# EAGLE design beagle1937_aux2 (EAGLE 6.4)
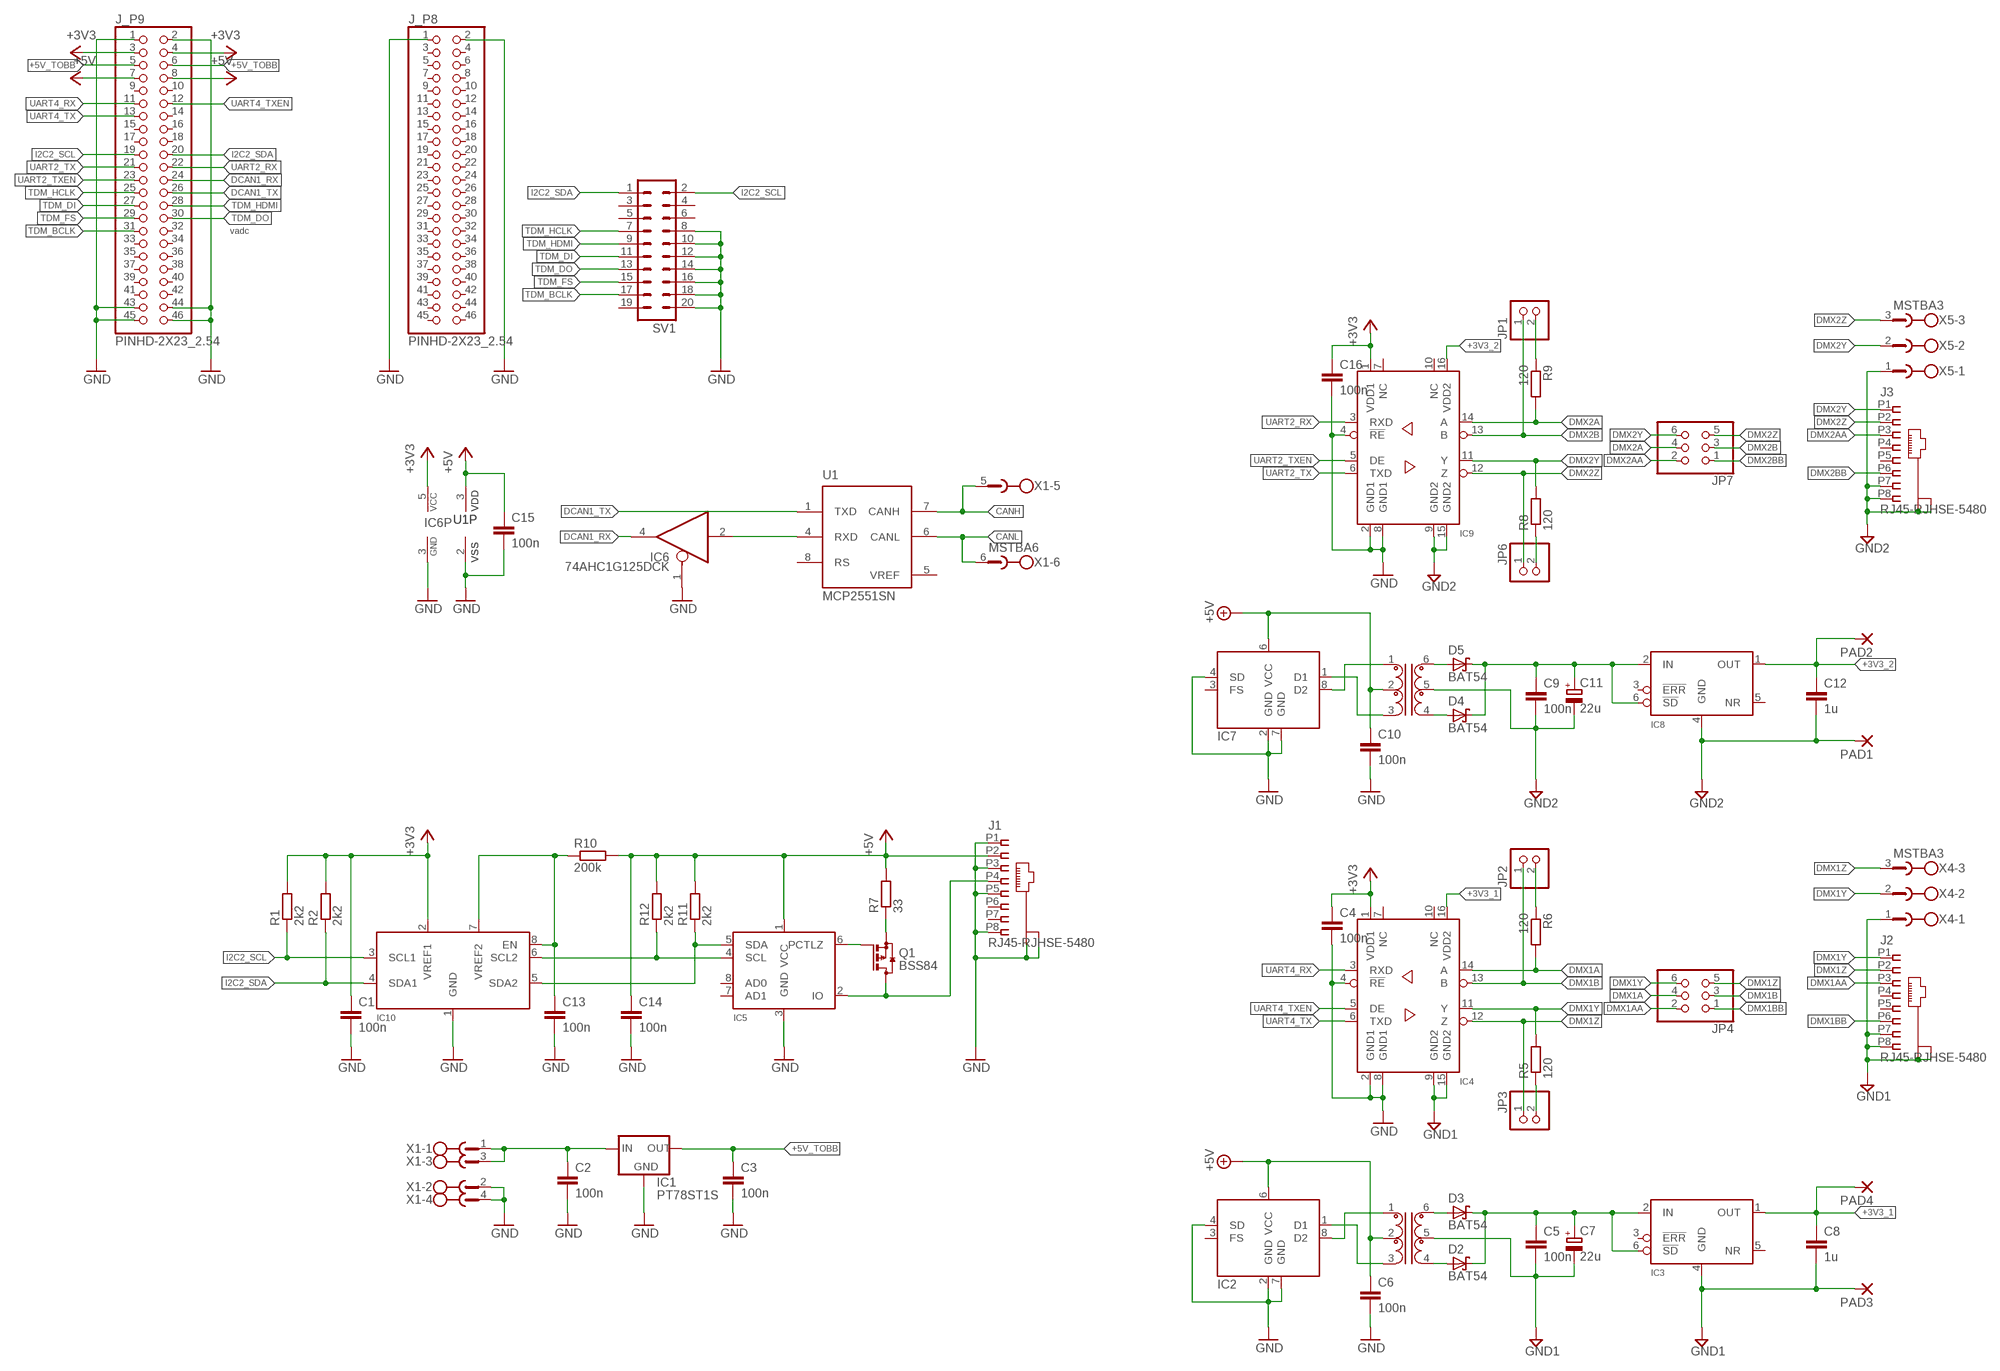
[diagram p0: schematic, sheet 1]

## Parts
C1  100n  C-EUC0603  [C0603]
C2  100n  C-EUC0603  [C0603]
C3  100n  C-EUC0603  [C0603]
C4  100n  C-EUC0603  [C0603]
C5  100n  C-EUC0603  [C0603]
C6  100n  C-EUC0603  [C0603]
C7  22u  CPOL-EUSMCA  [SMC_A]
C8  1u  C-EUC0603  [C0603]
C9  100n  C-EUC0603  [C0603]
C10  100n  C-EUC0603  [C0603]
C11  22u  CPOL-EUSMCA  [SMC_A]
C12  1u  C-EUC0603  [C0603]
C13  100n  C-EUC0603  [C0603]
C14  100n  C-EUC0603  [C0603]
C15  100n  C-EUC0603  [C0603]
C16  100n  C-EUC0603  [C0603]
D2  BAT54  [SOT23]
D3  BAT54  [SOT23]
D4  BAT54  [SOT23]
D5  BAT54  [SOT23]
IC1  PT78ST1S  [PT78ST100S]
IC2  MAX253CSA  [SO08]
IC3  ADP3330ART  [SOT23-6]
IC4  ADM2484EBRWZ  [SO16_XL]
IC5  DS2482S  [SO08]
IC6  74AHC1G125DCK  [SC70-5]
IC7  MAX253CSA  [SO08]
IC8  ADP3330ART  [SOT23-6]
IC9  ADM2484EBRWZ  [SO16_XL]
IC10  PCA9306D  [SO08]
J1  RJ45-RJHSE-5480  [RJHS-NOLEDS]
J2  RJ45-RJHSE-5480  [RJHS-NOLEDS]
J3  RJ45-RJHSE-5480  [RJHS-NOLEDS]
J_P8  PINHD-2X23_2.54  [2X23]
J_P9  PINHD-2X23_2.54  [2X23]
JP1  PINHD-1X2_2.54  [1X02]
JP2  PINHD-1X2_2.54  [1X02]
JP3  PINHD-1X2_2.54  [1X02]
JP4  PINHD-2X3_2.54  [2X03]
JP6  PINHD-1X2_2.54  [1X02]
JP7  PINHD-2X3_2.54  [2X03]
PAD1  SMD5  [SMD2,54-5,08]
PAD2  SMD5  [SMD2,54-5,08]
PAD3  SMD5  [SMD2,54-5,08]
PAD4  SMD5  [SMD2,54-5,08]
Q1  BSS84  [SOT23]
R1  2k2  R-EU_R0603  [R0603]
R2  2k2  R-EU_R0603  [R0603]
R5  120  R-EU_R0603  [R0603]
R6  120  R-EU_R0603  [R0603]
R7  33  R-EU_R0603  [R0603]
R8  120  R-EU_R0603  [R0603]
R9  120  R-EU_R0603  [R0603]
R10  200k  R-EU_R0603  [R0603]
R11  2k2  R-EU_R0603  [R0603]
R12  2k2  R-EU_R0603  [R0603]
SV1  ML20  [ML20]
T1  78253  [78253]
T2  78253  [78253]
U1  MCP2551SN  [SO-08]
X1  MSTBA6  [MSTBA6]
X4  MSTBA3  [MSTBA3]
X5  MSTBA3  [MSTBA3]

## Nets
1W: IC5.2(IO) J1.P4 Q1.3(D)
+3V3: C1.1 C4.1 C16.1 IC4.1(VDD1) IC6.5(VCC) IC9.1(VDD1) IC10.2(VREF1) J_P9.3 J_P9.4 R1.2 R2.2
+3V3_1: C8.1 IC3.1(OUT) IC4.16(VDD2) PAD4.1(P)
+3V3_2: C12.1 IC8.1(OUT) IC9.16(VDD2) PAD2.1(P)
+5V: C6.1 C10.1 C14.1 C15.1 IC2.6(VCC) IC5.1(VCC) IC7.6(VCC) J1.P2 J_P9.7 J_P9.8 R7.2 R10.2 R11.2 R12.2 T1.2 T2.2 U1.3(VDD)
+5V_1: C5.1 C7.+ D2.3(C) D3.3(C) IC3.2(IN) IC3.6(!SD)
+5V_2: C9.1 C11.+ D4.3(C) D5.3(C) IC8.2(IN) IC8.6(!SD)
+5V_TOBB: C3.1 IC1.3(OUT) J_P9.5 J_P9.6
+24V: C2.1 IC1.1(IN) X1.1 X1.3
CANH: U1.7(CANH) X1.5
CANL: U1.6(CANL) X1.6
DCAN1_RX: IC6.4(O) J_P9.24
DCAN1_TX: J_P9.26 U1.1(TXD)
DMX1A: IC4.14(A) JP4.4 R6.2
DMX1AA: J2.P3 JP4.2
DMX1B: IC4.13(B) JP2.1 JP4.3
DMX1BB: J2.P6 JP4.1
DMX1Y: IC4.11(Y) J2.P1 JP4.6 R5.2 X4.2
DMX1Z: IC4.12(Z) J2.P2 JP3.1 JP4.5 X4.3
DMX2A: IC9.14(A) JP7.4 R9.2
DMX2AA: J3.P3 JP7.2
DMX2B: IC9.13(B) JP1.1 JP7.3
DMX2BB: J3.P6 JP7.1
DMX2Y: IC9.11(Y) J3.P1 JP7.6 R8.2 X5.2
DMX2Z: IC9.12(Z) J3.P2 JP6.1 JP7.5 X5.3
GND: C1.2 C2.2 C3.2 C4.2 C6.2 C10.2 C13.2 C14.2 C15.2 C16.2 IC1.2(GND) IC2.2(GND) IC2.4(SD) IC2.7(GND) IC4.2(GND1) IC4.4(!RE) IC4.8(GND1) IC5.3(GND) IC6.1(OE) IC6.3(GND) IC7.2(GND) IC7.4(SD) IC7.7(GND) IC9.2(GND1) IC9.4(!RE) IC9.8(GND1) IC10.1(GND) J1.GND1(S1) J1.GND2(S2) J1.P1 J1.P3 J1.P5 J1.P8 J_P8.1 J_P8.2 J_P9.1 J_P9.2 J_P9.43 J_P9.44 J_P9.45 J_P9.46 SV1.8 SV1.10 SV1.12 SV1.14 SV1.16 SV1.18 SV1.20 U1.2(VSS) X1.2 X1.4
GND1: C5.2 C7.- C8.2 IC3.4(GND) IC4.9(GND2) IC4.15(GND2) J2.GND1(S1) J2.GND2(S2) J2.P7 J2.P8 PAD3.1(P) T1.5 X4.1
GND2: C9.2 C11.- C12.2 IC8.4(GND) IC9.9(GND2) IC9.15(GND2) J3.GND1(S1) J3.GND2(S2) J3.P7 J3.P8 PAD1.1(P) T2.5 X5.1
I2C2_SCL: IC10.3(SCL1) J_P9.19 R1.1 SV1.2
I2C2_SDA: IC10.4(SDA1) J_P9.20 R2.1 SV1.1
N$1: IC7.1(D1) T2.3
N$8: IC6.2(I) U1.4(RXD)
N$9: IC7.8(D2) T2.1
N$10: IC2.1(D1) T1.3
N$11: IC2.8(D2) T1.1
N$12: D2.1(A) T1.4
N$13: D3.1(A) T1.6
N$14: Q1.2(S) R7.1
N$15: JP3.2 R5.1
N$16: JP2.2 R6.1
N$17: D4.1(A) T2.4
N$18: D5.1(A) T2.6
N$19: JP6.2 R8.1
N$20: JP1.2 R9.1
N$21: C13.1 IC10.7(VREF2) IC10.8(EN) R10.1
N$22: IC5.4(SCL) IC10.6(SCL2) R12.1
N$23: IC5.5(SDA) IC10.5(SDA2) R11.1
PCTLZ: IC5.6(PCTLZ) Q1.1(G)
TDM_BCLK: J_P9.31 SV1.17
TDM_DI: J_P9.27 SV1.11
TDM_DO: J_P9.30 SV1.13
TDM_FS: J_P9.29 SV1.15
TDM_HCLK: J_P9.25 SV1.7
TDM_HDMI: J_P9.28 SV1.9
UART2_RX: IC9.3(RXD) J_P9.22
UART2_TX: IC9.6(TXD) J_P9.21
UART2_TXEN: IC9.5(DE) J_P9.23
UART4_RX: IC4.3(RXD) J_P9.11
UART4_TX: IC4.6(TXD) J_P9.13
UART4_TXEN: IC4.5(DE) J_P9.12
Unconnected: IC2.3(FS) IC3.3(!ERR) IC3.5(NR) IC4.7(NC) IC4.10(NC) IC5.7(AD1) IC5.8(AD0) IC7.3(FS) IC8.3(!ERR) IC8.5(NR) IC9.7(NC) IC9.10(NC) J1.P6 J1.P7 J2.P4 J2.P5 J3.P4 J3.P5 J_P8.3 J_P8.4 J_P8.5 J_P8.6 J_P8.7 J_P8.8 J_P8.9 J_P8.10 J_P8.11 J_P8.12 J_P8.13 J_P8.14 J_P8.15 J_P8.16 J_P8.17 J_P8.18 J_P8.19 J_P8.20 J_P8.21 J_P8.22 J_P8.23 J_P8.24 J_P8.25 J_P8.26 J_P8.27 J_P8.28 J_P8.29 J_P8.30 J_P8.31 J_P8.32 J_P8.33 J_P8.34 J_P8.35 J_P8.36 J_P8.37 J_P8.38 J_P8.39 J_P8.40 J_P8.41 J_P8.42 J_P8.43 J_P8.44 J_P8.45 J_P8.46 J_P9.9 J_P9.10 J_P9.14 J_P9.15 J_P9.16 J_P9.17 J_P9.18 J_P9.32 J_P9.33 J_P9.34 J_P9.35 J_P9.36 J_P9.37 J_P9.38 J_P9.39 J_P9.40 J_P9.41 J_P9.42 SV1.3 SV1.4 SV1.5 SV1.6 SV1.19 U1.8(RS)

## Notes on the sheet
- vadc

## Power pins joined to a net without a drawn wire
VREF: U1.5(VREF)

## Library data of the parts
C1-C6 C8-C10 C12-C16 = rcl:C-EU: CAPACITOR, European symbol
C7 C11 = rcl:CPOL-EU: POLARIZED CAPACITOR, European symbol
D2-D5 = diode:BAT54: Schottky Diodes
IC1 = equinox:PT78ST1**S: PT78ST1**S
IC2 IC7 = equinox:MAX253: Transformer Driver for Isolated RS-485 Interface
IC3 IC8 = equinox:ADP3330A: High Accuracy Ultralow IQ, 200 mA, SOT-23, anyCAPTM Low Dropout Regulator
IC4 IC9 = equinox:ADM2484E: 500 kbps, ESD Protected, Half-/Full-Duplex, iCoupler, Isolated RS-485 Transceiver
IC5 = equinox:DS2482: Single-Channel 1-Wire Master
IC6 = 74xx-little-us:74*1G125: Single Bus Buffer Gate with 3-State Output
IC10 = equinox:PCA9306: Dual bidirectional I2C-bus and SMBus voltage-level translator
J1-J3 = equinox:RJ45: RJ45
J_P8 J_P9 = pinhead-1:PINHD-2X23: PIN HEADER
JP1-JP3 JP6 = pinhead-1:PINHD-1X2: PIN HEADER
JP4 JP7 = pinhead-1:PINHD-2X3: PIN HEADER
PAD1-PAD4 = wirepad:SMD5: SMD PAD
Q1 = transistor-small-signal:BSS84: P-CHANNEL MOS FET
R1 R2 R5-R12 = rcl:R-EU_: RESISTOR, European symbol
SV1 = con-ml:ML20: HARTING; OC_FARNELL: unknown; OC_NEWARK: unknown
T1 T2 = equinox:78253: MAX253 Compatible Converter Transformers
U1 = microchip_can:MCP2551: High Speed CAN tranceiver
X1 = con-phoenix-508:MSTBA6: PHOENIX; MF: FARNELL; MPN: 1757284; OC_FARNELL: 3705213; OC_NEWARK: 71C4165
X4 X5 = con-phoenix-508:MSTBA3: PHOENIX; MF: FARNELL; MPN: 1757255; OC_FARNELL: 3705183; OC_NEWARK: 71C4162

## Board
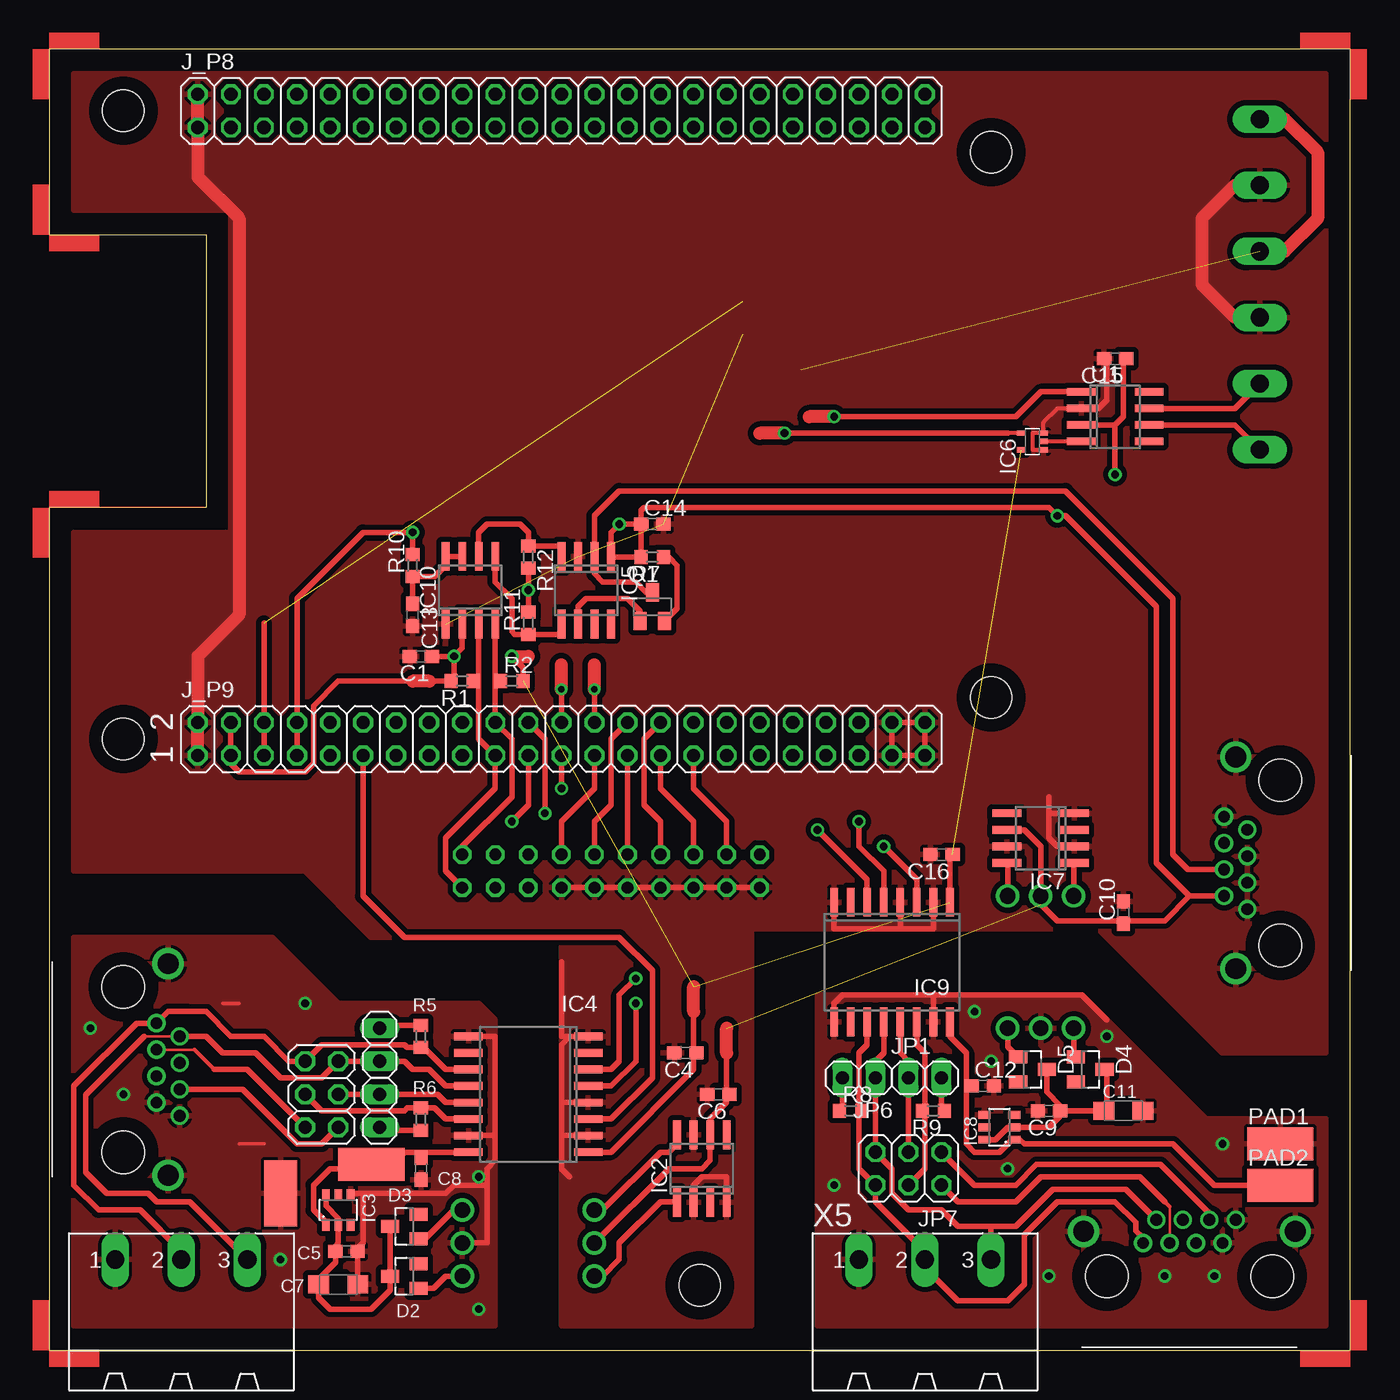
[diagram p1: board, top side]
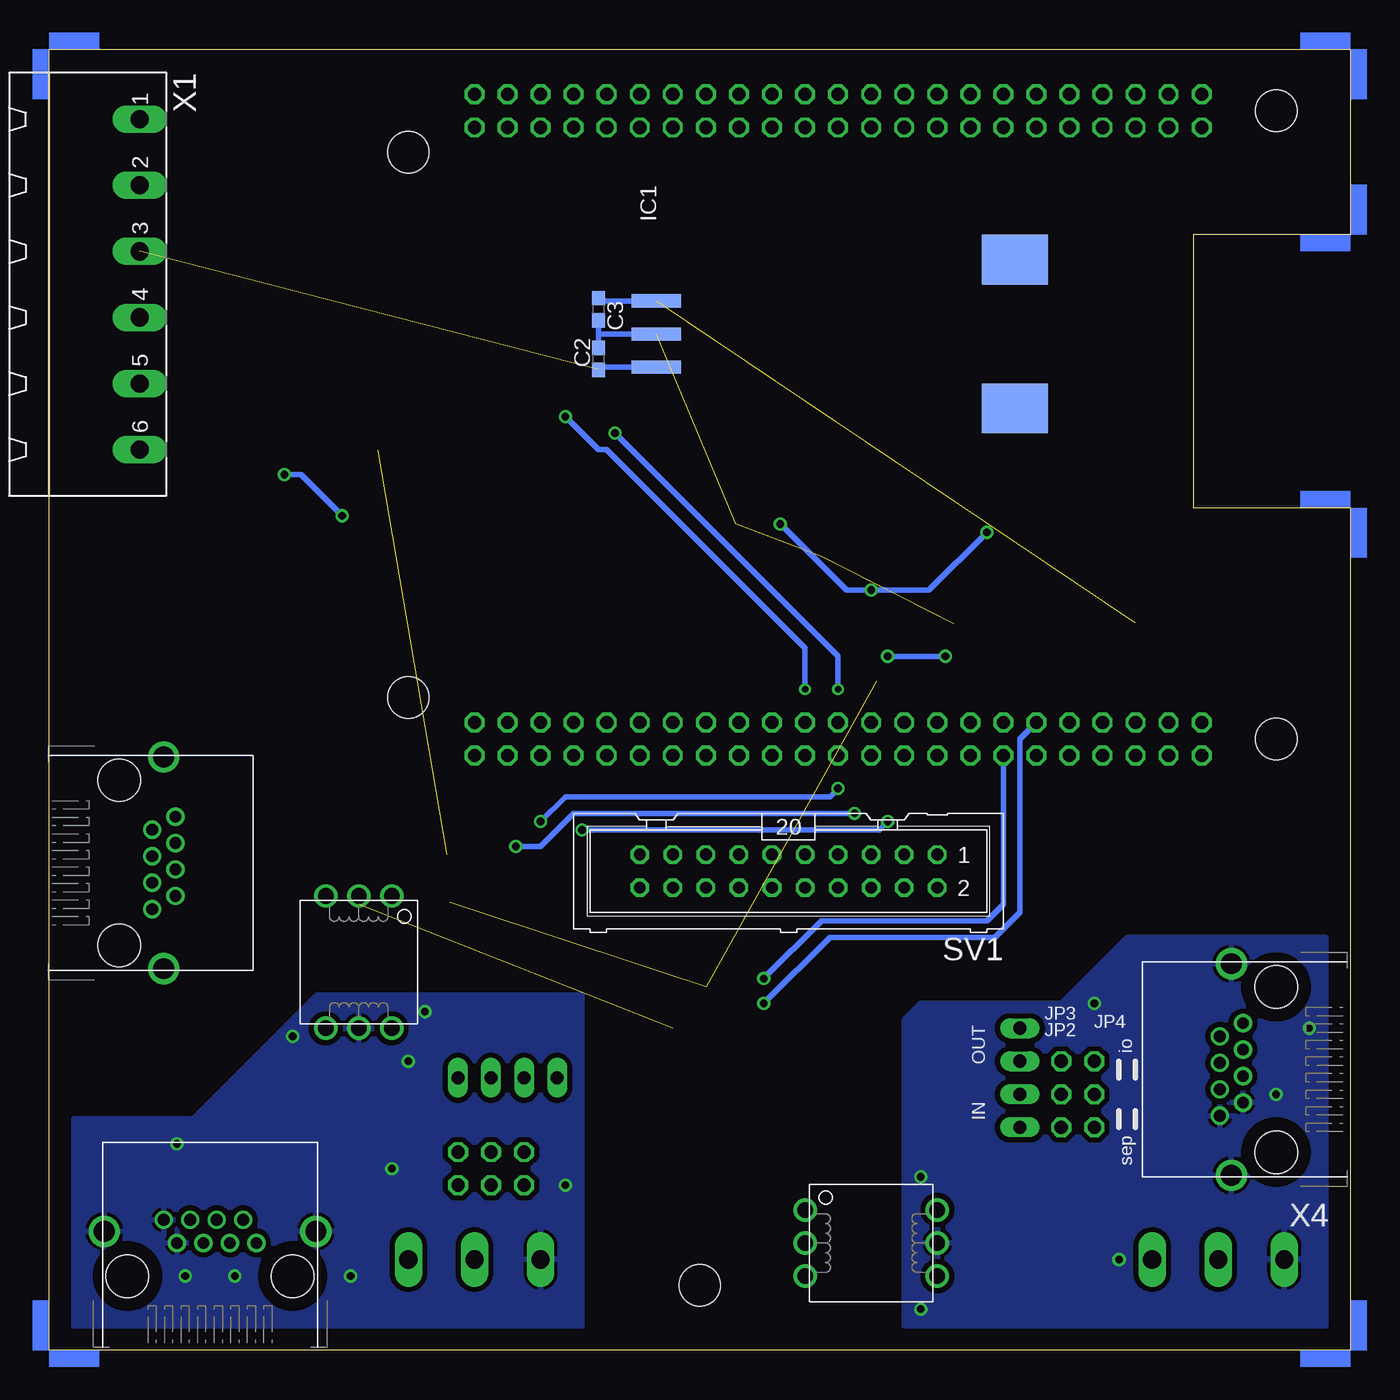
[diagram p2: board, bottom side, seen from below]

Size 100 x 100 mm. Coordinates in mm from the lower left corner, seen from the top.
Outline: 0,0 100,0 100,100 0,100 0,85.72 12.06,85.72 12.06,64.77 0,64.77 0,0
Copper layers (1*16): Top 0.035mm / dielectric 1.5mm / Bottom 0.035mm
Design rules "default": minimum track width 10mil, minimum drill 24mil, track to track 8mil, track to pad 8mil, pad to pad 8mil, via to via 8mil, smd to smd 8mil, copper to edge 40mil, drill to drill 8mil, minimum pad ring 10mil, minimum via ring 8mil, stop-mask expansion 4mil, vias tented up to drill 0mil, thermal gap 10mil
Holes 3.2 mm at 5.71,46.99 5.71,95.25 72.39,92.08 72.39,50.16 50,5
tRestrict: area 75.3,20.2 to 75.8,23; area 79.8,20.2 to 80.3,23; area 78.2,21.3 to 79.8,21.8; area 72.5,17.7 to 73.5,17.8; area 82,17.7 to 83.1,19.2; area 21.7,4.3 to 22.7,5.8; area 22.7,10.3 to 22.9,11.3; area 51.2,19.2 to 51.4,20.2; area 73.8,21.3 to 75.3,21.8; 9 lines

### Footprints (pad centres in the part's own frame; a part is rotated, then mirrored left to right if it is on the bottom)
C0603 = smd 1.1 x 1: 1 -0.85,0; 2 0.85,0
SMC_A = smd 1.6 x 1.4: + -1.5,0; - 1.5,0
SOT23 = smd 1 x 1.4: 1 -0.95,-1.1; 2 0.95,-1.1; 3 0,1.1
PT78ST100S = smd 1.016 x 3.81: 1 2.54,1.905; 2 0,1.905; 3 -2.54,1.905 | smd 3.81 x 5.08: MOUNT@@0 5.715,29.464; MOUNT@@1 -5.715,29.464
SO08 = smd 0.6 x 2.2: 1 -1.905,-2.6; 2 -0.635,-2.6; 3 0.635,-2.6; 4 1.905,-2.6; 5 1.905,2.6; 6 0.635,2.6; 7 -0.635,2.6; 8 -1.905,2.6
SOT23-6 = smd 0.6 x 0.9: 1 -0.95,-1.15; 2 0,-1.15; 3 0.95,-1.15; 4 0.95,1.15; 5 0,1.15; 6 -0.95,1.15
SO16_XL = smd 0.6 x 2.2: 1 -4.445,-4.6; 2 -3.175,-4.6; 3 -1.905,-4.6; 4 -0.635,-4.6; 5 0.635,-4.6; 6 1.905,-4.6; 7 3.175,-4.6; 8 4.445,-4.6; 9 4.445,4.6; 10 3.175,4.6; 11 1.905,4.6; 12 0.635,4.6; 13 -0.635,4.6; 14 -1.905,4.6; 15 -3.175,4.6; 16 -4.445,4.6
SC70-5 = smd 0.4 x 0.7: 1 -0.65,-0.85; 2 0,-0.85; 3 0.65,-0.85; 4 0.65,0.85; 5 -0.65,0.85
RJHS-NOLEDS = drill 1.6: GND1 -8.128,3.429; GND2 8.128,3.429 | drill 0.9: P1 3.556,2.54; P2 2.54,4.318; P3 1.524,2.54; P4 0.508,4.318; P5 -0.508,2.54; P6 -1.524,4.318; P7 -2.54,2.54; P8 -3.556,4.318 | hole 3.277: 6.35,0; -6.35,0
2X23 = drill 1.016 octagon: 1 -25.4,-1.27; 2 -25.4,1.27; 3 -22.86,-1.27; 4 -22.86,1.27; 5 -20.32,-1.27; 6 -20.32,1.27; 7 -17.78,-1.27; 8 -17.78,1.27; 9 -15.24,-1.27; 10 -15.24,1.27; 11 -12.7,-1.27; 12 -12.7,1.27; 13 -10.16,-1.27; 14 -10.16,1.27; 15 -7.62,-1.27; 16 -7.62,1.27; 17 -5.08,-1.27; 18 -5.08,1.27; 19 -2.54,-1.27; 20 -2.54,1.27; 21 0,-1.27; 22 0,1.27; 23 2.54,-1.27; 24 2.54,1.27; 25 5.08,-1.27; 26 5.08,1.27; 27 7.62,-1.27; 28 7.62,1.27; 29 10.16,-1.27; 30 10.16,1.27; 31 12.7,-1.27; 32 12.7,1.27; 33 15.24,-1.27; 34 15.24,1.27; 35 17.78,-1.27; 36 17.78,1.27; 37 20.32,-1.27; 38 20.32,1.27; 39 22.86,-1.27; 40 22.86,1.27; 41 25.4,-1.27; 42 25.4,1.27; 43 27.94,-1.27; 44 27.94,1.27; 45 30.48,-1.27; 46 30.48,1.27
1X02 = drill 1.016 long: 1 -1.27,0; 2 1.27,0
2X03 = drill 1.016 octagon: 1 -2.54,-1.27; 2 -2.54,1.27; 3 0,-1.27; 4 0,1.27; 5 2.54,-1.27; 6 2.54,1.27
SMD2,54-5,08 = smd 2.54 x 5.08: 1 0,0
R0603 = smd 1 x 1.1: 1 -0.85,0; 2 0.85,0
ML20 = drill 0.914 octagon: 1 -11.43,-1.27; 2 -11.43,1.27; 3 -8.89,-1.27; 4 -8.89,1.27; 5 -6.35,-1.27; 6 -6.35,1.27; 7 -3.81,-1.27; 8 -3.81,1.27; 9 -1.27,-1.27; 10 -1.27,1.27; 11 1.27,-1.27; 12 1.27,1.27; 13 3.81,-1.27; 14 3.81,1.27; 15 6.35,-1.27; 16 6.35,1.27; 17 8.89,-1.27; 18 8.89,1.27; 19 11.43,-1.27; 20 11.43,1.27
78253 = drill 1.2: 1 -5.08,2.54; 2 -5.08,0; 3 -5.08,-2.54; 4 5.08,-2.54; 5 5.08,0; 6 5.08,2.54
SO-08 = smd 0.6 x 2.2: 1 -1.905,-2.6; 2 -0.635,-2.6; 3 0.635,-2.6; 4 1.905,-2.6; 5 1.905,2.6; 6 0.635,2.6; 7 -0.635,2.6; 8 -1.905,2.6
MSTBA6 = drill 1.397 long: 1 -12.7,5.08; 2 -7.62,5.08; 3 -2.54,5.08; 4 2.54,5.08; 5 7.62,5.08; 6 12.7,5.08
MSTBA3 = drill 1.397 long: 1 -5.08,5.08; 2 0,5.08; 3 5.08,5.08

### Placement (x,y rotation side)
C1  28.57,53.34 180 top
C2  57.78,76.2 90 bottom
C3  57.78,80.01 270 bottom
C4  48.9,22.86 180 top
C5  22.86,7.62 0 top
C6  51.44,19.68 180 top
C7  22.23,5.08 0 top
C8  28.57,13.97 270 top
C9  76.83,18.41 180 top
C10  82.55,33.66 90 top
C11  82.55,18.41 0 top
C12  71.75,20.32 0 top
C13  27.94,56.52 270 top
C14  46.35,63.5 0 top
C15  81.92,76.2 180 top
C16  68.58,38.1 180 top
D2  27.3,5.71 90 top
D3  27.3,9.53 90 top
D4  80.01,21.59 270 top
D5  75.56,21.59 270 top
IC1  PT78ST1*S  [PT78ST100S]  55.24,78.11 270 bottom
IC2  50.16,13.97 0 top
IC3  22.23,10.79 0 top
IC4  36.83,19.68 90 top
IC5  41.27,58.42 180 top
IC6  75.56,69.85 90 top
IC7  76.2,39.37 90 top
IC8  73.03,17.14 90 top
IC9  64.77,29.84 180 top
IC10  32.38,58.42 0 top
J1  94.61,37.47 270 bottom
J2  5.71,21.59 90 bottom
J3  87.63,5.71 0 bottom
J_P8  36.83,95.25 0 top
J_P9  36.83,46.99 0 top
JP1  67.31,20.95 0 top
JP2  25.4,18.41 270 top
JP3  25.4,23.5 90 top
JP4  20.95,19.68 90 top
JP6  62.23,20.95 180 top
JP7  66.04,13.97 180 top
PAD1  94.61,15.88 270 top
PAD2  94.61,12.7 270 top
PAD3  17.78,12.06 0 top
PAD4  24.77,14.29 90 top
Q1  46.35,57.15 0 top
R1  31.75,51.44 180 top
R2  35.56,51.44 0 top
R5  28.57,24.13 270 top
R6  28.57,17.78 90 top
R7  46.35,60.96 180 top
R8  61.59,18.41 0 top
R9  67.94,18.41 180 top
R10  27.94,60.33 90 top
R11  36.83,55.88 90 top
R12  36.83,60.96 270 top
SV1  43.18,36.83 180 bottom
T1  36.83,8.26 0 bottom
T2  76.2,29.84 270 bottom
U1  81.92,71.75 270 top
U$1  [BBONE-CAPE]  not placed on the board
U$2  [ANGLE-SE1-16]  0,0 0 top
U$3  [ANGLE-SE1-16]  100,0 90 top
U$4  [ANGLE-SE1-16]  0,64.77 270 top
U$5  [ANGLE-SE1-16]  0,85.72 0 top
U$6  [ANGLE-SE1-16]  0,100 270 top
U$7  [ANGLE-SE1-16]  100,100 180 top
X1  98.11,81.92 270 bottom
X4  10.16,1.91 0 top
X5  67.31,1.91 0 top

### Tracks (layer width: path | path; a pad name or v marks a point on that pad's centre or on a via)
1W
  Top 0.406: Q1.3 45.89,58.25 45.09,59.05 42.55,59.05 41.91,59.69 IC5.2 41.91,64.14 43.81,66.04 78.11,66.04 86.36,57.78 86.36,38.1 87.5,36.96 J1.P4
+3V3  (via drill 0.6)  (3 unrouted)
  Top 0.406: J_P9.4 J_P9.3 13.97,45.09 14.61,44.45 19.68,44.45 20.32,45.09 20.32,49.53 22.23,51.44 27.94,51.44 | IC4.1 43.18,15.24 49.53,21.59 49.53,22.86 | 49.53,22.86 49.53,26.04 | IC10.2 31.75,53.98 v31.11,53.34 | C1.1 v31.11,53.34 | v31.11,53.34 31.11,51.44 R1.2 29.21,51.44 | R2.2 36.41,52.49 v35.56,53.34 | C4.1 49.53,22.86 | C16.1 69.22,38.1 IC9.1
  Top 1.016: v35.56,53.34 36.83,53.34 | 29.21,51.44 27.94,51.44 | 49.53,26.04 49.53,27.94
  Bottom 0.406: v31.11,53.34 v35.56,53.34
+3V3_1
  Top 0.406: IC3.1 21.27,9.84 20.32,10.79 20.32,12.7 21.59,13.97 24.77,13.97 | IC4.16 28.57,15.24 | 28.57,15.24 27.3,15.24 26.04,13.97 24.77,13.97 | C8.1 28.57,15.24 | PAD4.1 24.77,13.97
+3V3_2
  Top 0.406: IC9.16 69.22,24.13 70.48,22.86 70.48,20.32 | 70.48,20.32 70.48,15.88 71.12,15.24 73.03,15.24 73.98,16.2 IC8.1 74.61,16.2 74.93,15.88 86.36,15.88 89.53,12.7 PAD2.1 | C12.1 70.48,20.32
+5V  (via drill 0.6)  (1 unrouted)
  Top 0.406: 52.07,19.47 C6.1 52.07,19.68 | J_P9.7 J_P9.8 19.05,57.78 24.13,62.87 v27.94,62.87 R10.2 | U1.3 81.92,71.12 | 81.92,71.12 82.55,71.75 82.55,75.98 C15.1 | C14.1 R7.2 43.24,60.96 IC5.1 43.18,62.87 v43.81,63.5 C14.1 | IC7.6 74.93,40.01 76.2,38.73 T2.2 76.2,34.29 77.47,33.02 82.55,33.02 | 52.07,19.47 52.07,19.68 | 52.07,19.68 52.07,22.86 | J1.P2 87.63,34.92 | 87.63,34.92 85.72,33.02 82.55,33.02 | R12.2 v36.83,58.42 R11.2 | T1.2 47.62,13.97 50.16,13.97 50.8,14.61 IC2.6 50.8,17.78 52.07,19.05 52.07,19.47 | C10.1 82.55,33.02 | 87.63,34.92 85.09,37.47 85.09,57.15 78.11,64.14 v77.47,64.14 76.83,64.77 45.72,64.77 45.51,64.56 C14.1 | 81.92,71.12 v81.92,67.31
  Top 1.016: 52.07,22.86 52.07,24.77
  Bottom 0.406: v27.94,62.87 32.38,58.42 v36.83,58.42 38.73,58.42 v43.81,63.5 | v81.92,67.31 80.64,67.31 v77.47,64.14
+5V_1
  Top 0.406: D3.3 D2.3 26.2,4.62 24.77,3.17 21.59,3.17 20.73,4.04 C7.+ 20.73,5.49 22.01,6.77 C5.1 22.01,8.04 22.23,8.26 IC3.2 22.23,10.16 21.27,11.11 IC3.6
+5V_2
  Top 0.406: IC8.6 72.71,16.2 73.66,17.14 IC8.2 76.83,17.14 77.69,18 C9.1 | C9.1 C11.+ 81.28,18.41 81.28,21.42 D4.3 | D5.3 76.67,19.86 77.69,18.84 C9.1
+5V_TOBB  (1 unrouted)
  Top 0.406: J_P9.5 J_P9.6 16.51,55.88
  Bottom 0.406: IC1.3 57.57,80.64 C3.1
+24V  (1 unrouted)
  Top 1.016: X1.1 94.93,94.61 97.47,92.08 97.47,87 94.93,84.45 X1.3
  Bottom 0.406: IC1.1 57.57,75.56 C2.1
CANH
  Top 0.406: U1.7 91.12,72.39 X1.5
CANL
  Top 0.406: U1.6 91.12,71.12 X1.6
DCAN1_RX  (via drill 0.5, 0.6)
  Top 0.305: IC6.4 73.66,70.5 73.64,70.48 73.66,70.48
  Top 0.406: J_P9.24 v39.37,50.8 | v56.52,70.48 73.66,70.48
  Top 1.016: v56.52,70.48 54.61,70.48 | v39.37,50.8 39.37,52.7
  Bottom 0.406: v39.37,50.8 39.37,53.35 39.38,53.35 v56.52,70.48
DCAN1_TX  (via drill 0.5, 0.6)
  Top 0.406: U1.1 76.2,73.66 74.3,71.75 v60.33,71.75 | J_P9.26 v41.91,50.8
  Top 1.016: v60.33,71.75 58.42,71.75 | v41.91,50.8 41.91,52.7
  Bottom 0.406: v41.91,50.8 41.91,53.98 57.15,69.22 57.78,69.22 v60.33,71.75
DMX1A
  Top 0.406: IC4.14 30.48,17.78 29.63,18.63 R6.2 27.52,18.63 27.3,18.41 20.95,18.41 JP4.4
DMX1AA
  Top 0.203: J2.P3 11.18,23.11
  Top 0.305: 11.18,23.11 12.7,21.59
  Top 0.406: JP4.2 15.24,21.59 12.7,21.59
DMX1B
  Top 0.406: IC4.13 30.48,19.05 29.84,19.68 JP2.1 JP4.3
DMX1BB
  Top 0.406: JP4.1 20.95,15.88 19.05,15.88 14.86,20.07 J2.P6
DMX1Y
  Top 0.406: IC4.11 30.48,21.59 28.79,23.28 R5.2 27.52,23.28 27.3,23.5 20.95,23.5 JP4.6 18.41,22.23 16.51,24.13 13.97,24.13 12.06,26.04 9.14,26.04 J2.P1 6.73,25.15 1.91,20.32 1.91,12.7 3.81,10.79 6.99,10.79 10.16,7.62 X4.2
DMX1Z
  Top 0.203: J2.P2 7.3,24.13
  Top 0.406: IC4.12 30.48,20.32 29.21,21.59 27.94,21.59 27.3,22.23 JP3.1 JP4.5 20.95,20.95 17.78,20.95 15.88,22.86 13.34,22.86 12.06,24.13 J2.P2 | X4.3 10.79,11.43 8.26,11.43 7.62,12.06 4.45,12.06 2.81,13.7 2.81,19.63 7.3,24.13
DMX2A
  Top 0.406: IC9.14 66.67,23.5 67.31,22.86 67.31,18.63 R9.2 67.31,18.2 67.31,13.97 JP7.4
DMX2AA
  Top 0.203: J3.P3 86.11,11.05
  Top 0.305: 86.11,11.05 85.72,11.43
  Top 0.406: JP7.2 69.85,11.43 74.3,11.43 76.2,13.34 83.82,13.34 85.72,11.43
DMX2B
  Top 0.406: IC9.13 65.41,22.86 66.04,22.23 JP1.1 JP7.3
DMX2BB
  Top 0.406: JP7.1 71.12,12.7 74.3,12.7 75.88,14.29 85.41,14.29 89.15,10.54 J3.P6
DMX2Y
  Top 0.406: IC9.11 62.87,23.5 62.23,22.86 62.23,18.63 R8.2 62.23,18.2 62.23,13.97 JP7.6 63.5,11.43 67.31,7.62 X5.2 67.31,6.35 69.85,3.81 73.66,3.81 74.93,5.08 74.93,8.89 77.47,11.43 81.92,11.43 83.5,9.84 83.5,9.21 84.07,8.64 J3.P1
DMX2Z
  Top 0.406: IC9.12 64.14,22.86 63.5,22.23 JP6.1 JP7.5 64.77,13.97 64.77,12.06 66.04,10.79 68.58,10.79 69.85,9.53 72.39,9.53 | 72.39,9.53 X5.3 | 72.39,9.53 74.3,9.53 77.15,12.38 82.74,12.38 J3.P2
GND  (3 unrouted)
  Top 0.305: IC6.1 75.58,69.2 75.56,69.22 75.56,70.48 75.58,70.5 IC6.3 76.42,71.33 77.47,72.39 U1.2
  Top 0.406: C6.2 50.8,19.68 | IC2.2 49.53,12.7 50.16,13.34 52.07,13.34 IC2.4 | 39.37,19.05 39.37,23.5 40.01,24.13 IC4.8 39.37,24.13 39.37,29.84 | 39.37,19.05 39.37,16.51 | 39.37,16.51 IC4.2 | 40.01,13.34 39.37,13.97 39.37,16.51 | IC4.4 39.37,19.05 | 88.57,83.17 88.58,83.19 | U1.2 80.64,72.39 81.28,73.03 81.28,75.98 C15.2 | 28.09,55.82 C13.2 | IC7.2 77.47,38.73 76.83,39.37 76.83,41.27 | 76.83,41.27 76.83,42.55 | IC7.4 76.83,41.27 | 65.41,32.38 67.94,32.38 IC9.2 | IC9.4 65.41,32.38 | 65.41,32.38 60.33,32.38 IC9.8 | SV1.20 SV1.18 SV1.16 SV1.14 SV1.12 SV1.10 SV1.8 | J_P9.43 J_P9.45 J_P9.46 J_P9.44 J_P9.43
  Top 1.016: J_P9.1 J_P9.2 11.43,53.34 14.61,56.52 14.61,87 11.43,90.17 J_P8.1 J_P8.2 | X1.2 91.12,89.53 88.58,87 88.58,83.19 88.58,81.92 91.12,79.38 X1.4
  Bottom 0.406: IC1.2 57.78,78.11 | 57.78,78.11 C3.2 | C2.2 57.78,78.11
  pour Top (isolate 0.406): 98.11,22.86 90.17,22.86 80.64,32.38 53.98,32.38 53.98,1.91 39.37,1.91 39.37,31.75 24.77,31.75 19.68,36.83 1.91,36.83 1.91,62.87 13.97,62.87 13.97,87.63 1.91,87.63 1.91,98.11 98.11,98.11
GND1  (via drill 0.6)
  Top 0.254: 14.61,15.88 16.51,15.88 | 13.34,26.67 14.61,26.67
  Top 0.406: C7.- 23.71,5.09 C5.2 23.71,7.83 24.13,8.26 24.13,12.06 | 32.38,8.26 33.66,8.26 33.66,12.7 | 33.66,12.7 31.11,12.7 30.48,12.06 24.13,12.06 | 24.13,12.06 23.3,12.06 IC3.4 | IC4.9 34.29,24.13 34.29,16.51 | 34.29,16.51 IC4.15 | 33.66,12.7 33.66,13.97 34.29,14.61 34.29,16.51
  other vias: 33.02,3.17 33.02,13.34 19.68,26.67 3.17,24.77 5.71,19.68 17.78,6.99
  pour Top (isolate 0.406): 34.29,1.91 1.91,1.91 1.91,31.75 17.14,31.75 22.23,26.67 33.02,26.67 34.29,25.4
  pour Top: 11.43,12.7 16.51,12.7 16.51,16.51 13.97,19.05 11.43,19.05
  pour Top: 10.79,26.67 20.32,26.67 20.32,27.94 18.41,29.84 10.79,29.84
  pour Top: 1.91,1.78 17.14,1.78 17.14,4.45 1.91,4.45
  pour Bottom (isolate 0.406): 1.91,31.75 17.14,31.75 22.23,26.67 33.02,26.67 34.29,25.4 34.29,1.91 1.91,1.91
GND2  (via drill 0.6)
  Top 0.406: 67.94,27.3 60.96,27.3 60.33,26.67 IC9.9 | IC9.15 67.94,27.3 | 67.94,27.3 79.38,27.3 81.28,25.4
  other vias: 81.28,24.13 71.12,26.04 60.33,12.7 90.17,15.88 89.53,5.71 85.72,5.71 76.83,5.71 73.66,13.97 72.39,22.23
  pour Top (isolate 0.406): 59.05,27.3 79.38,27.3 88.9,17.78 98.11,17.78 98.11,1.91 59.05,1.91
  pour Bottom (isolate 0.406): 59.05,27.3 79.38,27.3 88.9,17.78 98.11,17.78 98.11,1.91 59.05,1.91
  pour Top: 59.05,1.78 76.83,1.78 76.83,4.45 75.25,4.45 73.98,3.17 69.22,3.17 67.94,4.45 59.05,4.45
I2C2_SCL
  Top 0.406: IC10.3 33.02,51.44 | 33.02,51.44 33.02,46.99 J_P9.19 34.29,43.18 30.48,39.37 30.48,36.83 SV1.2 | R1.1 33.02,51.44
I2C2_SDA
  Top 0.406: 34.29,51.44 J_P9.20 35.56,46.99 35.56,42.55 31.75,38.73 SV1.1 | 34.29,51.44 IC10.4 | R2.1 34.29,51.44
N$1
  Top 0.406: IC7.1 78.74,37.47 T2.3
N$8
  Top 0.305: U1.4 IC6.2
N$9
  Top 0.406: IC7.8 73.66,37.47 T2.1
N$10
  Top 0.406: T1.3 42.55,5.71 43.81,6.99 43.81,8.26 46.99,11.43 48.2,11.43 IC2.1
N$11
  Top 0.406: 48.2,16.51 IC2.8 48.26,15.88 47.62,15.24 46.99,15.24 42.55,10.79 T1.1
N$12
  Top 0.406: D2.1 29.53,4.76 30.48,5.71 T1.4
N$13
  Top 0.406: D3.1 28.89,8.57 31.11,10.79 T1.6
N$14
  Top 0.406: R7.1 47.62,60.96 48.26,60.33 48.26,57.01 Q1.2
N$15
  Top 0.406: R5.1 25.61,24.98 JP3.2
N$16
  Top 0.406: R6.1 25.61,16.93 JP2.2
N$17
  Top 0.406: T2.4 78.74,22.71 D4.1
N$18
  Top 0.406: T2.6 73.66,23.34 D5.1
N$19
  Top 0.406: R8.1 60.96,18.41 JP6.2
N$20
  Top 0.406: R9.1 68.58,18.41 JP1.2
N$21
  Top 0.406: IC10.7 IC10.8 30.48,60.33 29.63,59.48 R10.1 C13.1
N$22
  Top 0.406: IC10.6 33.02,62.87 33.66,63.5 36.2,63.5 36.83,62.87 R12.1 39.16,61.81 39.37,61.59 IC5.4
N$23
  Top 0.406: IC10.5 34.29,59.05 35.56,57.78 35.56,55.24 35.77,55.03 R11.1 39.16,55.03 39.37,55.24 IC5.5
PCTLZ
  Top 0.406: Q1.1 45.41,56.83 44.45,57.78 41.27,57.78 40.64,57.15 IC5.6
TDM_BCLK
  Top 0.406: J_P9.31 49.53,43.18 52.07,40.64 SV1.17
TDM_DI
  Top 0.406: J_P9.27 SV1.11
TDM_DO
  Top 0.406: J_P9.30 45.72,46.99 45.72,41.91 46.99,40.64 SV1.13
TDM_FS
  Top 0.406: J_P9.29 46.99,43.18 49.53,40.64 SV1.15
TDM_HCLK
  Top 0.406: J_P9.25 41.91,43.18 39.37,40.64 SV1.7
TDM_HDMI
  Top 0.406: J_P9.28 43.18,46.99 43.18,41.91 41.91,40.64 SV1.9
UART2_RX  (via drill 0.6)
  Top 0.406: IC9.3 66.67,36.2 v64.14,38.73 | J_P9.22 38.1,46.99 v38.1,41.27
  Bottom 0.406: v64.14,38.73 62.23,38.73 59.69,41.27 v38.1,41.27
UART2_TX  (via drill 0.6)
  Top 0.406: IC9.6 62.87,36.2 v59.05,40.01 | J_P9.21 36.83,41.91 v35.56,40.64
  Bottom 0.406: v35.56,40.64 36.2,40.01 v59.05,40.01
UART2_TXEN  (via drill 0.6)
  Top 0.406: IC9.5 64.14,36.83 62.23,38.73 v62.23,40.64 | J_P9.23 v39.37,43.18
  Bottom 0.406: v39.37,43.18 40.01,42.55 60.33,42.55 v62.23,40.64
UART4_RX
  Top 0.406: IC4.3 43.18,17.78 46.35,20.95 46.35,29.21 43.81,31.75 27.3,31.75 24.13,34.92 J_P9.11
UART4_TX  (via drill 0.6)
  Top 0.406: IC4.6 43.18,21.59 43.81,22.23 43.81,27.3 v45.09,28.57
  Bottom 0.406: v45.09,28.57 40.64,33.02 27.94,33.02 26.67,34.29 J_P9.13
UART4_TXEN  (via drill 0.6)
  Top 0.406: IC4.5 43.18,20.32 45.09,22.23 v45.09,26.67
  Bottom 0.406: v45.09,26.67 40.01,31.75 27.3,31.75 25.4,33.66 25.4,46.99 J_P9.12
(copper drawn outside any net)
  shapes: Top circle x6

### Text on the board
tNames: 2 | 1
bNames: io | OUT | IN | sep
tRestrict: bid/out | in | DMX | GND | D | !d | GND | D | !d
Document: \! mechanical conflicts \! / do not move VR without check
refdoc: reset | leds | power | pwr led | bat | usb | DC jack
